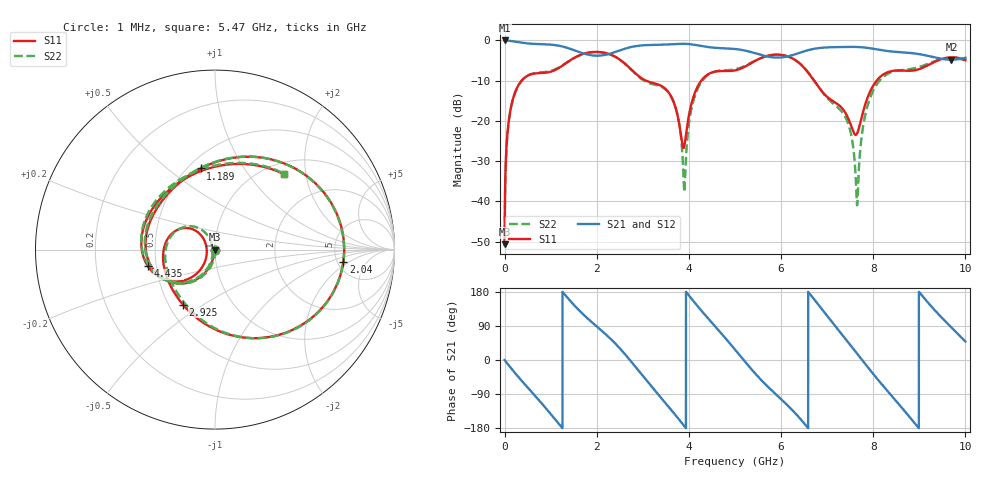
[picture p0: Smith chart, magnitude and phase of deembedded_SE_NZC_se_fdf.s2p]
# GHz S MA R 50
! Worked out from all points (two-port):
!   10000 points, 1 MHz to 10 GHz, reference 50 ohm
!   highest |S21| = 0.00 dB at 1 MHz (marker M1); lowest = -4.8 dB at 9.696 GHz (marker M2)
!   |S21| within 3 dB of the highest: 2.369 GHz to 5.386 GHz (3.017 GHz wide, 77.8 % of centre); 6.421 GHz to 8.688 GHz (2.266 GHz wide, 30 % of centre)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
!   lowest |S11| = -50.6 dB at 1 MHz (marker M3), VSWR 1.01, Z = 49.7 - j0.124 ohm
!   |S11| at or under -10 dB: start of sweep to 368.7 MHz; 3.071 GHz to 4.269 GHz (1.198 GHz wide, 32.7 % of centre); 6.715 GHz to 8.074 GHz (1.359 GHz wide, 18.4 % of centre)
!   |S22| runs from -51.1 to -2.9 dB; largest |S21 - S12| = 1.8e-15
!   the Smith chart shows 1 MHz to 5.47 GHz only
!   S11 on the Smith chart (normalised r, x): 1 MHz: 0.99, -0.00; 1.189 GHz: 0.58, +0.66; 2.04 GHz: 5.65, -1.57; 2.925 GHz: 0.59, -0.41; 4.435 GHz: 0.45, -0.10; 5.47 GHz: 1.22, +1.52
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0.001  0.002941 -155.0  0.9999 -0.2  0.9999 -0.2  0.002773 -24.3
0.081  0.08993 -106.5  0.9929 -12.6  0.9929 -12.6  0.08655 -102.3
0.239  0.2349 -128.6  0.9647 -36.1  0.9647 -36.1  0.2304 -127.1
0.706  0.3912 169.1  0.9031 -100.5  0.9031 -100.5  0.397 167.9
1.189  0.459 100.0  0.8576 -170.1  0.8576 -170.1  0.465 99.0
1.668  0.6684 34.2  0.702 125.0  0.702 125.0  0.6663 34.5
2.04  0.7184 -5.4  0.6471 84.4  0.6471 84.4  0.7179 -5.4
2.925  0.3547 -120.2  0.8615 -30.8  0.8615 -30.8  0.3482 -117.4
3.334  0.2832 177.4  0.8828 -90.9  0.8828 -90.9  0.2748 -179.8
3.9  0.04854 -160.6  0.9091 -174.3  0.9091 -174.3  0.01305 -177.2
4.435  0.3851 -166.1  0.8251 107.2  0.8251 107.2  0.3799 -166.2
5.001  0.4243 118.7  0.7828 27.3  0.7828 27.3  0.4379 114.2
5.47  0.5703 47.2  0.6852 -39.9  0.6852 -39.9  0.5722 47.8
6.145  0.6345 -27.7  0.6339 -120.1  0.6339 -120.1  0.6329 -27.9
6.667  0.3456 -95.8  0.7767 168.0  0.7767 168.0  0.35 -92.9
7.162  0.1714 178.2  0.8259 91.6  0.8259 91.6  0.1586 -169.0
7.648  0.06945 -164.1  0.8296 17.2  0.8296 17.2  0.009006 -171.6
7.881  0.1972 -137.5  0.8079 -18.9  0.8079 -18.9  0.1569 -114.5
8.334  0.4069 -178.1  0.7359 -85.2  0.7359 -85.2  0.3897 179.3
8.957  0.4329 96.7  0.6819 -175.1  0.6819 -175.1  0.4606 89.0
9.696  0.6177 -5.6  0.5766 86.2  0.5766 86.2  0.6063 -3.0
10  0.5679 -36.8  0.6086 48.8  0.6086 48.8  0.5614 -36.9
